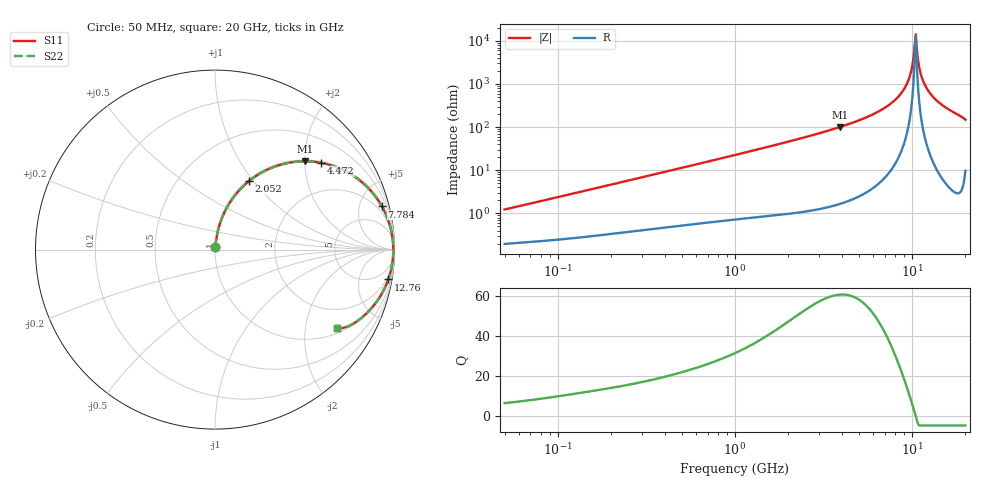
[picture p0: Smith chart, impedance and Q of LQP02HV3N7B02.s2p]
!Murata Part Number: LQP02HV3N7B02
!These Parameters are Measured in Series Mode Connection
!  o--[Z]--o
!Port1  Port2
!  o-------o
!Freq. Start=50[MHz] Stop=20[GHz], 401[Steps]
# Hz S RI R 50
!Freq.(Hz) S11(Real) S11(Imag) S21(Real) S21(Imag) S12(Real) S12(Imag) S22(Real) S22(Imag)
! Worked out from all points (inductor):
!   401 points, 50 MHz to 20 GHz, reference 50 ohm
!   read as one part in series: L = 3.84 nH near 51.52 MHz
!   highest Q = 60.8 at 3.908 GHz (marker M1), where L = 4.09 nH
!   self-resonance near 10.35 GHz
!   S11 on the Smith chart (normalised r, x): 50 MHz: 1.00, +0.02; 2.052 GHz: 1.02, +0.95; 4.472 GHz: 1.04, +2.42; 7.784 GHz: 1.23, +7.68; 12.76 GHz: 1, -12; 20 GHz: 1.20, -2.97
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5e7  0.0021 0.0121  0.9979 -0.0121  0.9979 -0.0121  0.0021 0.0121
1.364002e8  0.0038 0.0319  0.9962 -0.0319  0.9962 -0.0319  0.0038 0.0319
3.721004e8  0.0116 0.0837  0.9884 -0.0837  0.9884 -0.0837  0.0116 0.0837
1e9  0.0547 0.2119  0.9453 -0.2119  0.9453 -0.2119  0.0547 0.2119
2.05233e9  0.1884 0.3807  0.8116 -0.3807  0.8116 -0.3807  0.1884 0.3807
2.728004e9  0.2994 0.449  0.7006 -0.449  0.7006 -0.449  0.2994 0.449
3.908127e9  0.5024 0.4918  0.4976 -0.4918  0.4976 -0.4918  0.5024 0.4918
4.472136e9  0.5926 0.4831  0.4074 -0.4831  0.4074 -0.4831  0.5926 0.4831
5.944466e9  0.7854 0.4011  0.2146 -0.4011  0.2146 -0.4011  0.7854 0.4011
7.442007e9  0.9108 0.2719  0.0892 -0.2719  0.0892 -0.2719  0.9108 0.2719
7.784049e9  0.9302 0.2401  0.0698 -0.2401  0.0698 -0.2401  0.9302 0.2401
8.644534e9  0.9663 0.16  0.0337 -0.16  0.0337 -0.16  0.9663 0.16
9.316812e9  0.9831 0.0989  0.0169 -0.0989  0.0169 -0.0989  0.9831 0.0989
9.892087e9  0.9909 0.0484  0.00907 -0.0484  0.00907 -0.0484  0.9909 0.0484
1.019291e10  0.9929 0.0229  0.00714 -0.0229  0.00714 -0.0229  0.9929 0.0229
1.050288e10  0.9935 -0.00269  0.00652 0.00269  0.00652 0.00269  0.9935 -0.00269
1.066139e10  0.9933 -0.0155  0.00671 0.0155  0.00671 0.0155  0.9933 -0.0155
1.115139e10  0.9907 -0.0539  0.00928 0.0539  0.00928 0.0539  0.9907 -0.0539
1.149051e10  0.9874 -0.0793  0.0126 0.0793  0.0126 0.0793  0.9874 -0.0793
1.276073e10  0.9654 -0.166  0.0346 0.166  0.0346 0.166  0.9654 -0.166
1.527346e10  0.8934 -0.2998  0.1066 0.2998  0.1066 0.2998  0.8934 -0.2998
2e10  0.6775 -0.4356  0.3225 0.4356  0.3225 0.4356  0.6775 -0.4356
